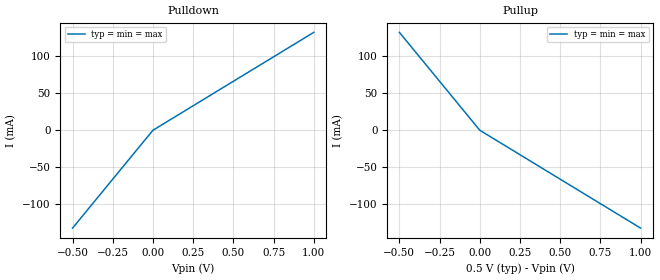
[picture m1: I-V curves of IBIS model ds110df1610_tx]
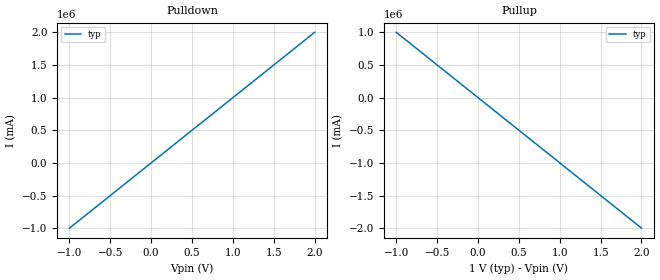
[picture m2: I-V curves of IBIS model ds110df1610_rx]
|Texas Instruments Incorporated
|16 channel retimer with integrated signal conditioning which includes
|an input Continuous-Time Linear Equalizer (CTLE),
|clock and data recovery (CDR)
|and transmit driver on each channel.
| Marketing part#   Voltage Range   Package-type   #pins
| D1xxDF1610   +2.375 to +2.625   FCBGA   196
[IBIS Ver]   5.0
[File Name]  ds110df1610.ibs
[File Rev]   1.0
[Component]  ds110df1610
[Manufacturer] Texas Instruments
[Disclaimer]
 This product is designed as an aid for customers of Texas Instruments.
 No warranties, either expressed or implied, with respect to this third
 party software (if any) or with respect to its fitness for any
 particular purpose is claimed by Texas Instruments or the author. The
 software (if any) is provided solely on an "as is" basis. The entire
 risk as to its quality and performance is with the customer
[Copyright] (C) Copyright 2013 Texas Instruments Incorporated.
   All rights reserved.
[Package]
R_pkg  0.0   NA   NA
L_pkg  0.0   NA   NA
C_pkg  0.0   NA   NA
[Pin]   signal_name   model_name   R_pin L_pin  C_pin
1p   Tx_p   ds110df1610_tx
1n   Tx_n   ds110df1610_tx
2p   Rx_p   ds110df1610_rx
2n   Rx_n   ds110df1610_rx
[Diff_Pin] inv_pin vdiff tdelay_typ tdelay_min tdelay_max
2p   2n   NA   NA   NA   NA
1p   1n   NA   NA   NA   NA
[Repeater_Pin]
2p 1p
| Models and submodels in the file (2): ds110df1610_tx (Output), ds110df1610_rx (Input)
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[Model] ds110df1610_tx
Model_type Output
C_comp 0p 0p 0p
Cref = 0
Vref = 0.5
Rref = 50
Vmeas = 0.5
[Temperature_Range] 25 125 0
[Voltage Range] 0.5 0.5 0.5
[Algorithmic Model]
Executable Windows_VisualC++ExpressEdition9.0.30729_32  ds110df1610_tx.dll ds110df1610_tx.ami
Executable Linux_gcc4.6.1_64 ds110df1610_tx_x64.so ds110df1610_tx.ami
[End Algorithmic Model]
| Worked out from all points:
|   slope of the pulldown table from 0 to 0.075 V, typ, clamps not added: 7.58 ohm
|   slope of the pullup table from 0 to 0.075 V, typ, clamps not added: 7.58 ohm
[Pulldown]
-500mV    -132mA     -132mA     -132mA
0V        0A         0A         0A
1V        132mA      132mA      132mA
[Pullup]
-500mV    132mA      132mA      132mA
0V        0A         0A         0A
1V        -132mA     -132mA     -132mA
[GND Clamp]
-500mV    0A         0A         0A
0V        0A         0A         0A
1V        0A         0A         0A
[Power Clamp]
-500mV    0A         0A         0A
0V        0A         0A         0A
1V        0A         0A         0A
[Ramp]
dV/dt_r 0.3/40p 0.3/40p 0.3/40p
dV/dt_f 0.3/40p 0.3/40p 0.3/40p
[Model] ds110df1610_rx
Model_type Input
C_comp 0p 0p 0p
Vinl = 0.3
Vinh = 0.7
[Temperature_Range] 25 125 0
[Voltage Range] 1.0 1.0 1.0
[Algorithmic Model]
Executable Windows_VisualC++ExpressEdition9.0.30729_32 ds110df1610_rx.dll ds110df1610_rx.ami
Executable Linux_gcc4.6.1_64 ds110df1610_rx_x64.so ds110df1610_rx.ami
[End Algorithmic Model]
[Ramp]
|   typ   min   max
dV/dt_r   0.8/1.0ps   NA   NA
dV/dt_f   0.8/1.0ps   NA   NA
R_load = 0.001ohm
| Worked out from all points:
|   slope of the pulldown table from 0 to 0.15 V, typ, clamps not added: 1 mohm
|   slope of the pullup table from 0 to 0.15 V, typ, clamps not added: 1 mohm
[Pulldown]
|Voltage I(typ)   I(min)   I(max)
-1V       -1kA       NA         NA
0V        0A         NA         NA
2V        2kA        NA         NA
[Pullup]
-1V       1kA        NA         NA
0V        0A         NA         NA
2V        -2kA       NA         NA
[GND Clamp]
-1V       0A         0A         0A
0V        0A         0A         0A
2V        0A         0A         0A
[Power Clamp]
-1V       0A         0A         0A
0V        0A         0A         0A
2V        0A         0A         0A
